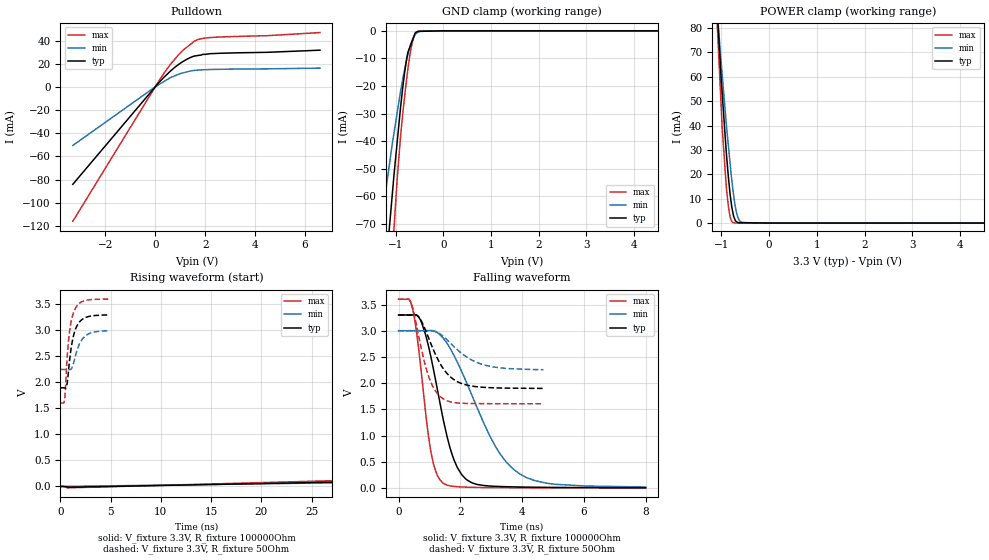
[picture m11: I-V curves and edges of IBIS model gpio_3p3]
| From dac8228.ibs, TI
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|   gpio_3p3 Model
[Model]   gpio_3p3
Model_type   I/O_open_drain
Polarity   Non-Inverting
Enable   Active-Low
Vinl = 0.6
Vinh = 2.3
Vmeas = 1.65
Vref = 3.3
Cref = 10pF
Rref = 100000
|   typ   min   max
|   (nom PVT)   (Fast PVT)   (slow PVT)
|C_comp from frequency method(F=50MHz)
|Average
C_comp   8.636e-12   7.116e-12   1.008e-11
|ON state : BUFFER OUTPUT TURNED LOW
|C_comp   8.804e-12   7.277e-12   1.026e-11
|OFF state: BUFFER IN HIGH IMPEDANCE
|C_comp   8.467e-12   6.956e-12   9.902e-12
|C_comp from L-C Tank method(L=1nH)
|Average
|C_comp   7.915e-12   6.670e-12   9.147e-12
|ON state : BUFFER OUTPUT TURNED LOW
|Resonant Frequency(Hz)   1.780e+09   1.930e+09   1.660e+09
|C_comp   8.003e-12   6.807e-12   9.201e-12
|OFF state: BUFFER IN HIGH IMPEDANCE
|Resonant Frequency(Hz)   1.800e+09   1.970e+09   1.670e+09
|C_comp   7.826e-12   6.533e-12   9.092e-12
| Where nom  PVT is Nominal Process,  3.3V,  33C
|   Fast PVT is Strong Process,   3.6V,  -40C
|   Slow PVT is Weak Process,   3V,  113C
[Voltage Range]   3.3   3   3.6
|Ambient Temperature   25   105   -40
|Junction Temperature
[Temperature Range]   33   113   -40
[Pullup Reference]   3.3   3   3.6
[Pulldown Reference]   0   0   0
[Power Clamp Reference]   3.3   3   3.6
[GND Clamp Reference]   0   0   0
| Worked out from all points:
|   slope of the pulldown table from 0 to 0.495 V, typ, clamps not added: 44 ohm
|   GND clamp passes 1 mA (typ) near -0.60 V on its own axis
|   POWER clamp passes 1 mA (typ) near -0.71 V on its own axis
|   falling waveform, V_fixture 3.3V, R_fixture 100000Ohm: 20-80 % time 725ps typ, 1.43ns min, 436ps max; typ from 3.3 V to 0.003 V
|   rising waveform, V_fixture 3.3V, R_fixture 100000Ohm: 20-80 % time 1.23us typ, 1.47us min, 1.01us max; typ from 0.001 V to 3.3 V
|   falling waveform, V_fixture 3.3V, R_fixture 50Ohm: 20-80 % time 710ps typ, 972ps min, 507ps max; typ from 3.3 V to 1.9 V
|   rising waveform, V_fixture 3.3V, R_fixture 50Ohm: 20-80 % time 708ps typ, 889ps min, 569ps max; typ from 1.9 V to 3.3 V
[Pulldown]
|   Voltage   I(typ)   I(min)   I(max)
-3.3V     -84.11mA   -50.56mA   -116mA
18mV      443.3uA    274.6uA    641.4uA
273.6mV   6.576mA    3.631mA    9.304mA
633.6mV   14.12mA    8.199mA    20.06mA
939.6mV   19.39mA    10.93mA    27.83mA
1.247V    23.62mA    12.83mA    33.99mA
1.566V    26.63mA    14.23mA    39.43mA
1.814V    27.44mA    14.64mA    41.5mA
2.203V    28.63mA    14.99mA    42.59mA
4.5V      29.86mA    15.58mA    44.23mA
6.6V      31.7mA     16.21mA    46.9mA
[GND Clamp]
|   Voltage   I(typ)   I(min)   I(max)
-3.3V     -572.7mA   -387.4mA   -802.2mA
-1.361V   -118.9mA   -77.73mA   -170.9mA
-1.272V   -100mA     -65.91mA   -143mA
-1.184V   -81.73mA   -55mA      -115.6mA
-1.071V   -59.2mA    -40.91mA   -81.77mA
-1.036V   -52.29mA   -37.09mA   -71.86mA
-896.4mV  -27.44mA   -21.78mA   -37.88mA
-811.8mV  -14.96mA   -13.98mA   -23.71mA
-738mV    -7.483mA   -8.126mA   -12.99mA
-655.2mV  -3.679mA   -3.589mA   -4.387mA
-537.9mV  -215.9uA   -600.8uA   -323.7uA
6.6V      0A         0A         0A
[POWER Clamp]
|   Voltage   I(typ)   I(min)   I(max)
-3.3V     869.3mA    734.6mA    1.044A
-1.084V   85.81mA    86.41mA    79.97mA
-1.032V   68.16mA    72.24mA    58.91mA
-982.8mV  52.97mA    60.65mA    38.83mA
-896.4mV  28.7mA     40.32mA    14.56mA
-853.2mV  18.73mA    31.56mA    6.771mA
-817.2mV  11.76mA    24.27mA    2.531mA
-756mV    3.952mA    13.19mA    210.4uA
-687mV    641.4uA    4.545mA    38.04uA
-651mV    146.4uA    2.075mA    32.51uA
-573mV    128.8uA    253uA      20.54uA
6.6V      0A         0A         0A
[Ramp]
R_load = 100000
|   typ   min   max
dV/dt_r   1.97809/1.23136e-06   1.796/1.46732e-06   2.15905/1.00462e-06
dV/dt_f   1.97921/7.27305e-10   1.7988/1.45405e-09   2.15938/4.41656e-10
[Falling Waveform]
V_fixture = 3.3V
V_fixture_min = 3V
V_fixture_max = 3.6V
R_fixture = 100000Ohm
|   Time   V(typ)   V(min)   V(max)
0s        3.3V       3V         3.6V
444ps     3.301V     3V         3.447V
742ps     3.161V     3V         2.182V
1.044ns   2.51V      3.002V     705.3mV
1.45ns    1.297V     2.855V     88.05mV
1.79ns    542.7mV    2.533V     28.73mV
2.172ns   172.7mV    2.05V      15.13mV
3.108ns   30.9mV     821.4mV    5.404mV
3.916ns   17.36mV    269mV      2.781mV
7.998ns   2.988mV    17.76mV    1.029mV
[Rising Waveform]
V_fixture = 3.3V
V_fixture_min = 3V
V_fixture_max = 3.6V
R_fixture = 100000Ohm
|   Time   V(typ)   V(min)   V(max)
0s        1.294mV    1.958mV    1.007mV
165.8ns   576.4mV    432.5mV    782mV
309.5ns   1.012V     774.2mV    1.331V
472.7ns   1.418V     1.108V     1.813V
648.3ns   1.765V     1.408V     2.202V
1.091us   2.361V     1.955V     2.819V
1.674us   2.788V     2.382V     3.212V
2.443us   3.055V     2.677V     3.435V
3.709us   3.223V     2.882V     3.557V
8us       3.298V     2.995V     3.599V
[Falling Waveform]
V_fixture = 3.3V
V_fixture_min = 3V
V_fixture_max = 3.6V
R_fixture = 50Ohm
|   Time   V(typ)   V(min)   V(max)
0s        3.3V       3V         3.6V
392ps     3.3V       3V         3.554V
488ps     3.302V     3V         3.366V
648ps     3.268V     3V         2.915V
940ps     2.913V     3.001V     2.191V
1.116ns   2.652V     2.998V     1.931V
1.376ns   2.342V     2.924V     1.73V
1.848ns   2.046V     2.667V     1.625V
2.648ns   1.924V     2.369V     1.609V
4.688ns   1.899V     2.256V     1.606V
[Rising Waveform]
V_fixture = 3.3V
V_fixture_min = 3V
V_fixture_max = 3.6V
R_fixture = 50Ohm
|   Time   V(typ)   V(min)   V(max)
0s        1.896V     2.249V     1.605V
404ps     1.894V     2.249V     1.652V
484ps     1.892V     2.249V     1.835V
648ps     1.962V     2.248V     2.416V
852ps     2.315V     2.244V     2.891V
1.1ns     2.701V     2.266V     3.201V
1.408ns   2.971V     2.447V     3.392V
1.892ns   3.16V      2.738V     3.52V
2.524ns   3.248V     2.9V       3.575V
4.828ns   3.296V     2.993V     3.599V
